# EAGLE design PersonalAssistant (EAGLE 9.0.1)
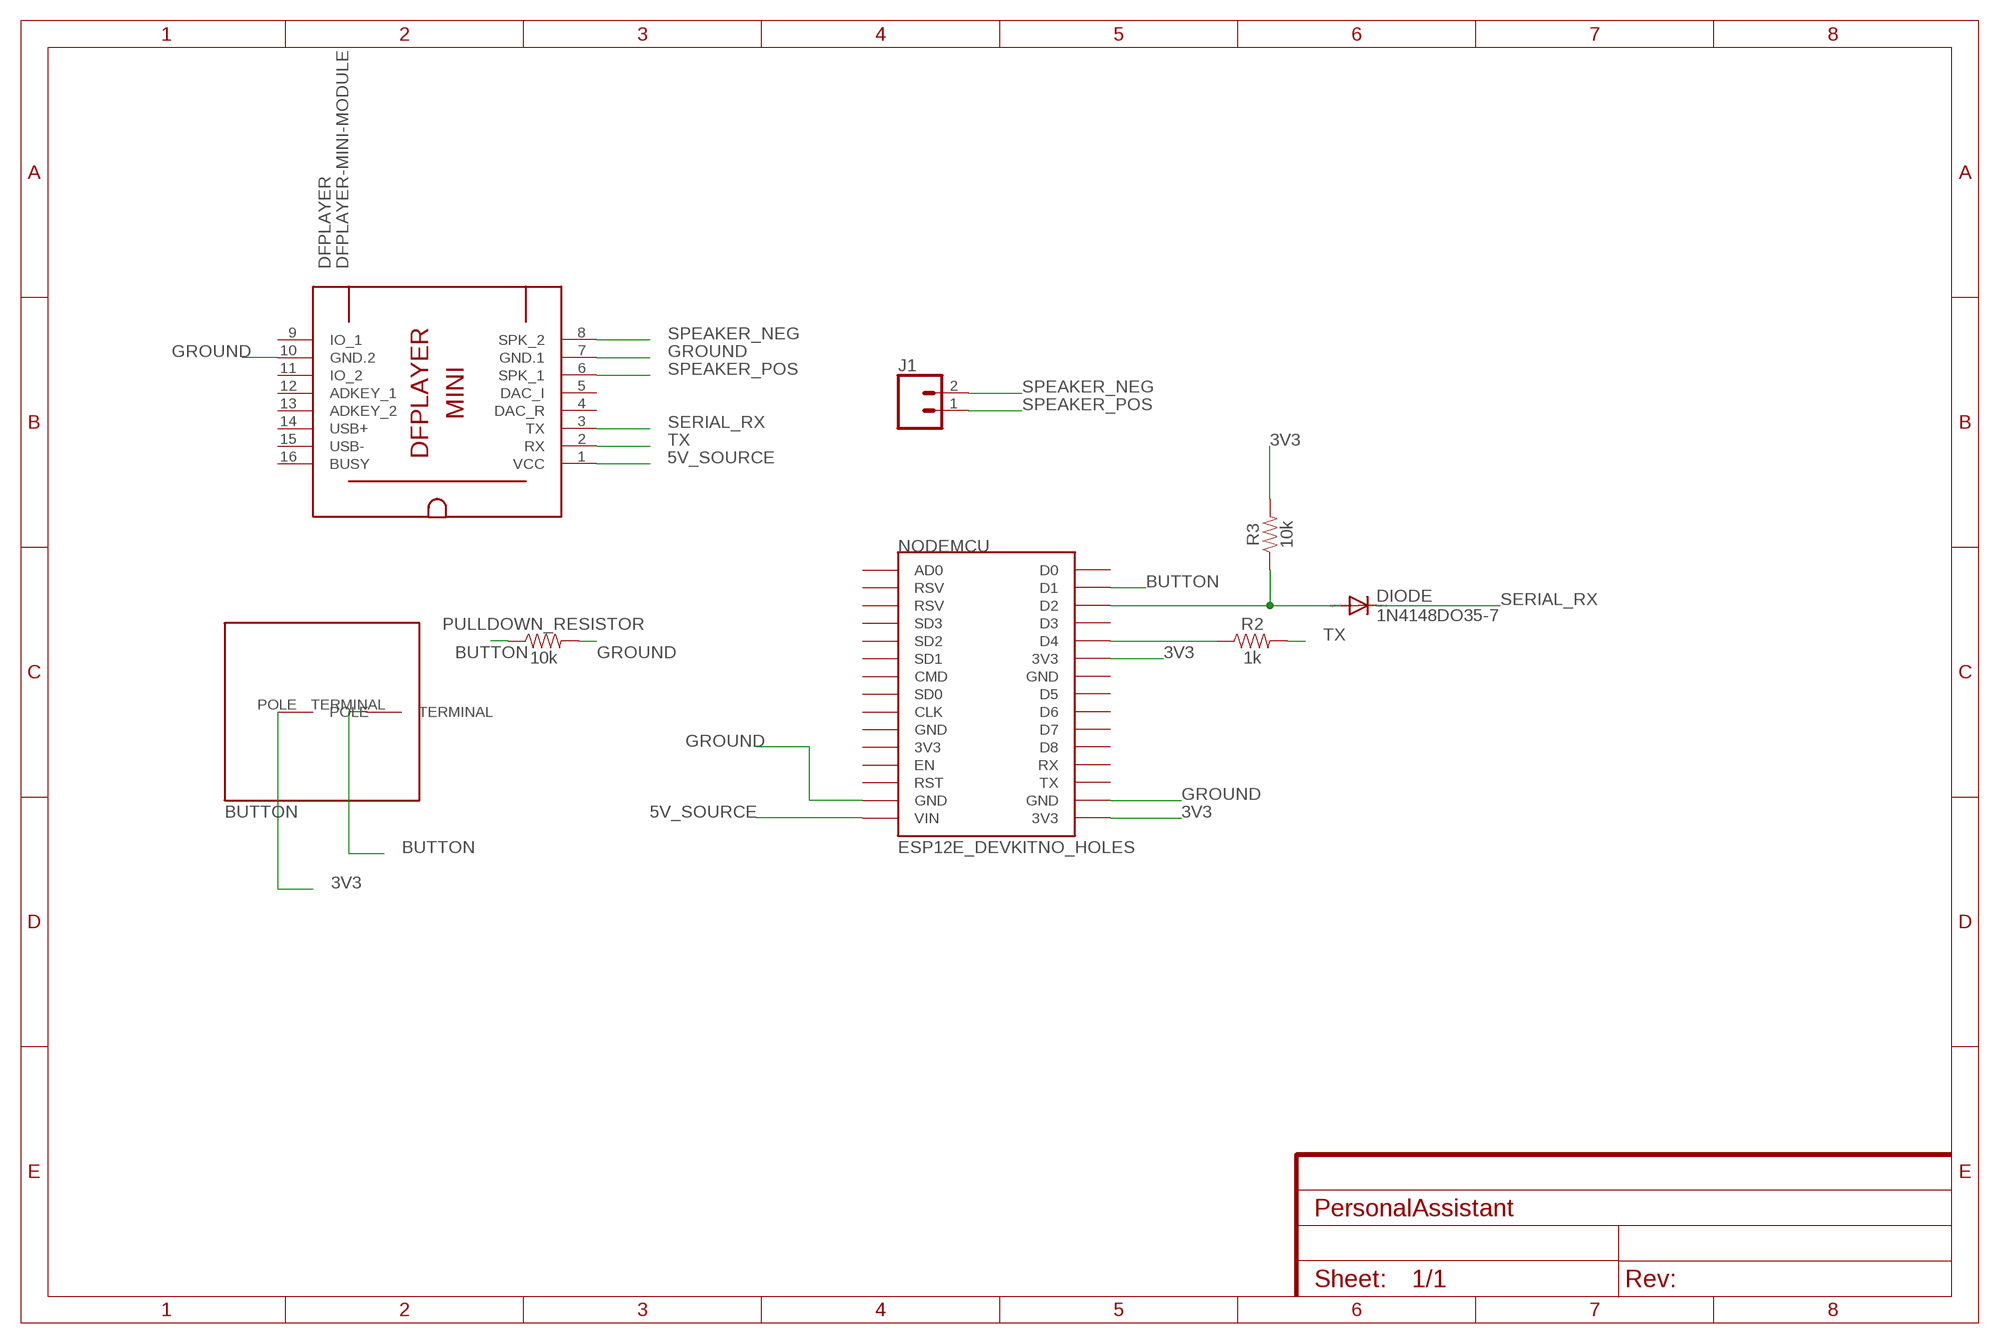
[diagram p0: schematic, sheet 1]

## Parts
BUTTON  SPST_MOMENTARY_BUTTON  [SPST_MOMENTRAY_BUTTON]
DFPLAYER  DFPLAYER-MINI-MODULE  [DFPLAYER-MINI-MODULE]
DIODE  1N4148DO35-7  [DO35-7]
J1  CONN_02  [1X02]
NODEMCU  ESP12E_DEVKITNO_HOLES  [ESP12E_DEVKIT]
PULLDOWN_RESISTOR  10k  10KOHM-HORIZ-1/4W-1%  [AXIAL-0.3]
R2  1k  10KOHM-HORIZ-1/4W-1%  [AXIAL-0.3]
R3  10k  10KOHM-HORIZ-1/4W-1%  [AXIAL-0.3]

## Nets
3V3: BUTTON.POLE NODEMCU.3V3@1(3V3) NODEMCU.3V3@2(3V3) R3.P$2
5V_SOURCE: DFPLAYER.1(VCC) NODEMCU.VIN
BUTTON: BUTTON.TERMINAL NODEMCU.D1 PULLDOWN_RESISTOR.P$1
GROUND: DFPLAYER.7(GND.1) DFPLAYER.10(GND.2) NODEMCU.GND@1(GND) NODEMCU.GND@3(GND) PULLDOWN_RESISTOR.P$2
N$1: NODEMCU.D4 R2.P$1
N$2: DIODE.A NODEMCU.D2 R3.P$1
SERIAL_RX: DFPLAYER.3(TX) DIODE.C
SPEAKER_NEG: DFPLAYER.8(SPK_2) J1.2
SPEAKER_POS: DFPLAYER.6(SPK_1) J1.1
TX: DFPLAYER.2(RX) R2.P$2
Unconnected: DFPLAYER.4(DAC_R) DFPLAYER.5(DAC_I) DFPLAYER.9(IO_1) DFPLAYER.11(IO_2) DFPLAYER.12(ADKEY_1) DFPLAYER.13(ADKEY_2) DFPLAYER.14(USB+) DFPLAYER.15(USB-) DFPLAYER.16(BUSY) NODEMCU.3V3@0(3V3) NODEMCU.AD0 NODEMCU.CLK NODEMCU.CMD NODEMCU.D0 NODEMCU.D3 NODEMCU.D5 NODEMCU.D6 NODEMCU.D7 NODEMCU.D8 NODEMCU.EN NODEMCU.GND@0(GND) NODEMCU.GND@2(GND) NODEMCU.RST NODEMCU.RSV@0(RSV) NODEMCU.RSV@1(RSV) NODEMCU.RX NODEMCU.SD0 NODEMCU.SD1 NODEMCU.SD2 NODEMCU.SD3 NODEMCU.TX

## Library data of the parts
BUTTON = spst_momentary_button:SPST_MOMENTARY_BUTTON
DFPLAYER = diy-modules:DFPLAYER-MINI-MODULE: DFPlayer Mini - MP3 player module based on YX5200 chip More details available here: https://www.dfrobot.com/wiki/index.php/DFPlayer_Mini_SKU:DFR0299 Click here to find device on ebay.com
DIODE = diode:1N4148: DIODE
J1 = SparkFun-Connectors:CONN_02: Multi connection point. Often used as Generic Header-pin footprint for 0.1 inch spaced/style header connections
NODEMCU = ESP12E_DEVKIT:ESP12E_DEVKIT: ESP12E DEVKIT BOARD
PULLDOWN_RESISTOR R3 = SparkFun-Resistors:10KOHM: 10kΩ resistor; PROD_ID: RES-12183
R2 = SparkFun-Resistors:10KOHM: 10kΩ resistor; PROD_ID: RES-12183; VALUE: 10k

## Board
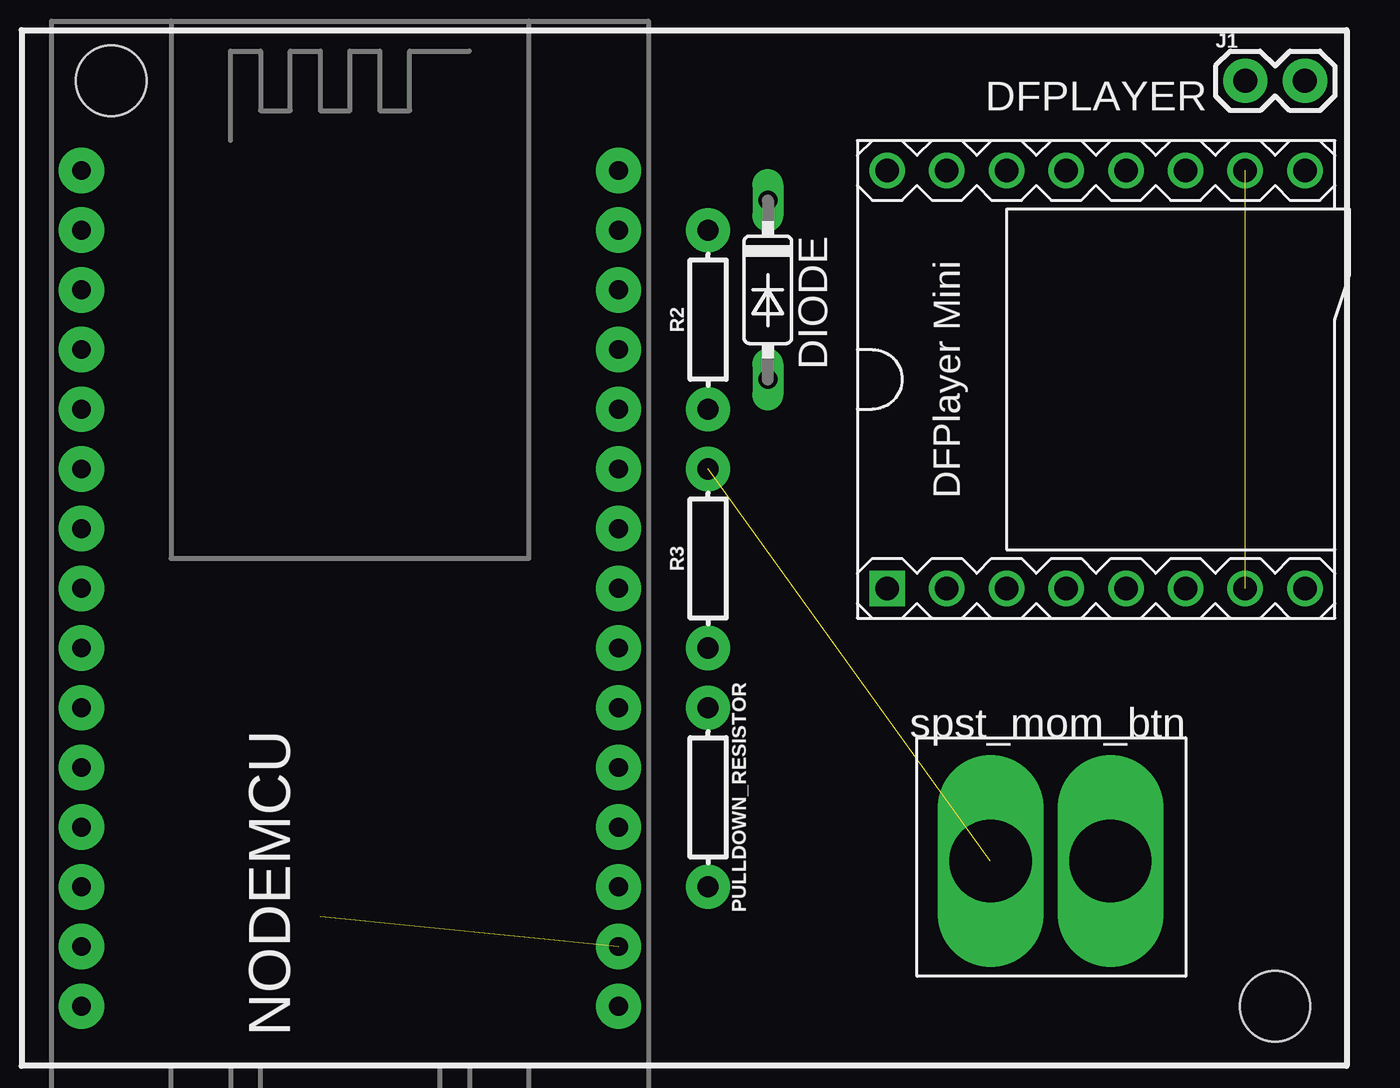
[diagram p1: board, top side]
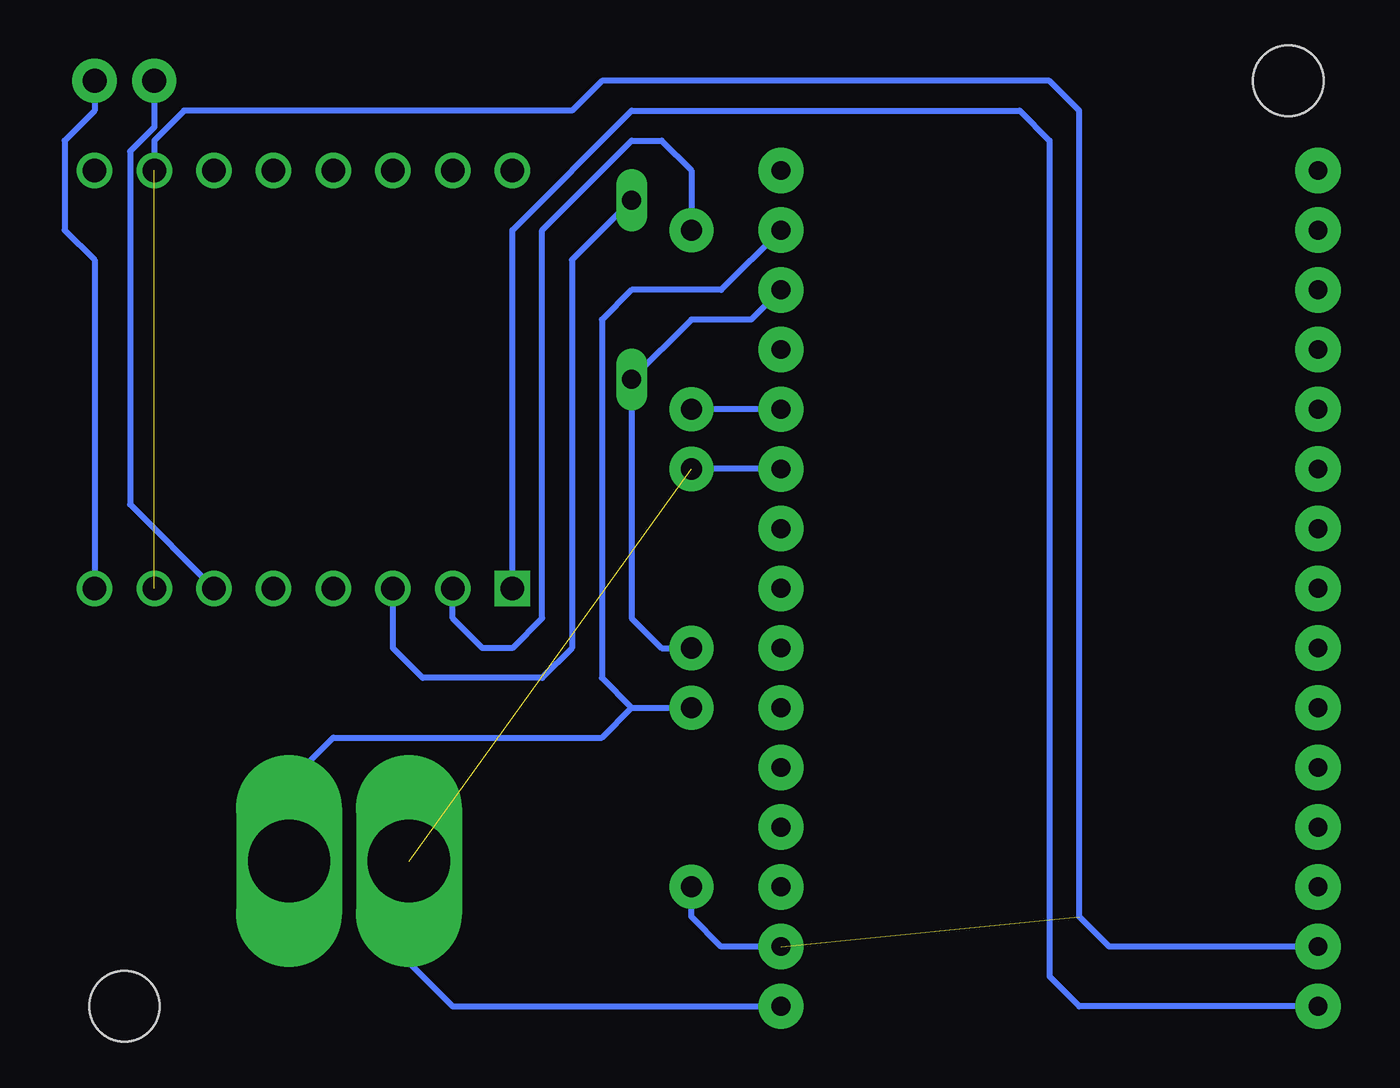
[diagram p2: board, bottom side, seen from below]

No outline drawn. Coordinates in mm, seen from the top.
Copper layers (1*16): Top 0.035mm / dielectric 1.5mm / Bottom 0.035mm
Design rules "default": minimum track width 6mil, minimum drill 0.35mm, track to track 6mil, track to pad 6mil, pad to pad 6mil, via to via 6mil, smd to smd 6mil, copper to edge 40mil, drill to drill 6mil, minimum pad ring 10mil, minimum via ring 8mil, stop-mask expansion 4mil, vias tented up to drill 0mil, thermal gap 10mil
Holes 3 mm at 13.97,44.45 63.5,5.08

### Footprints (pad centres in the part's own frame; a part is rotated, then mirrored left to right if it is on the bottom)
SPST_MOMENTRAY_BUTTON = drill 3.5 long: POLE 8.3,5.25; TERMINAL 3.2,5.25
DFPLAYER-MINI-MODULE = drill 1 square: 1 -8.89,-8.89 | drill 1: 2 -6.35,-8.89; 3 -3.81,-8.89; 4 -1.27,-8.89; 5 1.27,-8.89; 6 3.81,-8.89; 7 6.35,-8.89; 8 8.89,-8.89; 9 8.89,8.89; 10 6.35,8.89; 11 3.81,8.89; 12 1.27,8.89; 13 -1.27,8.89; 14 -3.81,8.89; 15 -6.35,8.89; 16 -8.89,8.89
DO35-7 = drill 0.813 long: A 3.81,0; C -3.81,0
1X02 = drill 1.016 pad 1.88: 1 0,0; 2 2.54,0
ESP12E_DEVKIT = drill 0.8 pad 1.93: 3V3@0 -11.43,-7.62; 3V3@1 11.43,5.08; 3V3@2 11.43,-17.78; AD0 -11.43,17.78; CLK -11.43,-2.54; CMD -11.43,2.54; D0 11.43,17.78; D1 11.43,15.24; D2 11.43,12.7; D3 11.43,10.16; D4 11.43,7.62; D5 11.43,0; D6 11.43,-2.54; D7 11.43,-5.08; D8 11.43,-7.62; EN -11.43,-10.16; GND@0 -11.43,-5.08; GND@1 -11.43,-15.24; GND@2 11.43,2.54; GND@3 11.43,-15.24; RST -11.43,-12.7; RSV@0 -11.43,15.24; RSV@1 -11.43,12.7; RX 11.43,-10.16; SD0 -11.43,0; SD1 -11.43,5.08; SD2 -11.43,7.62; SD3 -11.43,10.16; TX 11.43,-12.7; VIN -11.43,-17.78
AXIAL-0.3 = drill 0.9 pad 1.88: P$1 -3.81,0; P$2 3.81,0

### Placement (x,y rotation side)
BUTTON  59.69,16.51 180 top
DFPLAYER  55.88,31.75 0 top
DIODE  41.91,35.56 270 top
J1  62.23,44.45 0 top
NODEMCU  24.13,22.86 0 top
PULLDOWN_RESISTOR  39.37,13.97 270 top
R2  39.37,34.29 90 top
R3  39.37,24.13 90 top

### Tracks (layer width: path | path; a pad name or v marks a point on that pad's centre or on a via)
3V3  (1 unrouted)
  Bottom 0.254: NODEMCU.3V3@1 R3.P$2 | NODEMCU.3V3@2 49.53,5.08 51.39,6.94 BUTTON.POLE
5V_SOURCE
  Bottom 0.254: NODEMCU.VIN 22.86,5.08 24.13,6.35 24.13,41.91 25.4,43.18 41.91,43.18 46.99,38.1 DFPLAYER.1
BUTTON
  Bottom 0.254: NODEMCU.D1 38.1,35.56 41.91,35.56 43.18,34.29 43.18,19.05 41.91,17.78 | 41.91,17.78 PULLDOWN_RESISTOR.P$1 | 41.91,17.78 43.18,16.51 54.61,16.51 56.49,14.63 BUTTON.TERMINAL
GROUND  (2 unrouted)
  Bottom 0.254: NODEMCU.GND@3 38.1,7.62 39.37,8.89 PULLDOWN_RESISTOR.P$2 | NODEMCU.GND@1 21.59,7.62 22.86,8.89 22.86,43.18 24.13,44.45 43.18,44.45 44.45,43.18 60.96,43.18 62.23,41.91 DFPLAYER.10
N$1
  Bottom 0.254: NODEMCU.D4 R2.P$1
N$2
  Bottom 0.254: NODEMCU.D2 36.83,34.29 39.37,34.29 DIODE.A 41.91,21.59 40.64,20.32 R3.P$1
SERIAL_RX
  Bottom 0.254: DIODE.C 44.45,36.83 44.45,20.32 45.72,19.05 50.8,19.05 52.07,20.32 DFPLAYER.3
SPEAKER_NEG
  Bottom 0.254: J1.2 64.77,43.18 66.04,41.91 66.04,38.1 64.77,36.83 DFPLAYER.8
SPEAKER_POS
  Bottom 0.254: J1.1 62.23,42.48 63.26,41.45 63.26,26.43 DFPLAYER.6
TX
  Bottom 0.254: R2.P$2 39.37,40.64 40.64,41.91 41.91,41.91 45.72,38.1 45.72,21.59 46.99,20.32 48.26,20.32 49.53,21.59 DFPLAYER.2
